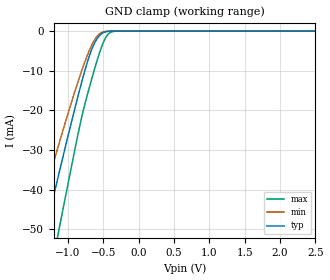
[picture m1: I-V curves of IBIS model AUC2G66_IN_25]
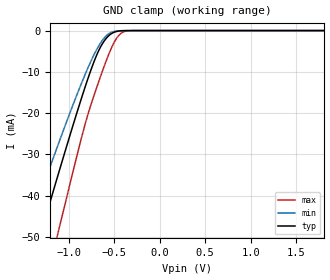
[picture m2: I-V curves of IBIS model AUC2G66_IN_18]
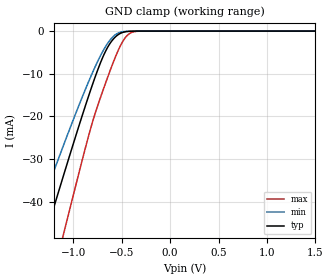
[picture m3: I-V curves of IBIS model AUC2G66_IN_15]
| TEXAS INSTRUMENTS INCORPORATED
| Standard Linear and Logic Group
| IBIS Model of SN74AUC2G66
| DUAL BILATERAL ANALOG SWITCH
| This file contains package information for the following:
|  SOT 8-pin (DCT) package as [Component] AUC2G66_DCT
|  TSSOP 8-pin (DCU) package as [Component] AUC2G66_DCU
|  NanoStar WCSP 8-pin (YEP) package as [Component] AUC2G66_YEP
|  NanoFree WCSP 8-pin (YZP) package as [Component] AUC2G66_YZP
| This device can be powered at the following Vccs:
|  2.5 volt Vcc
|  1.8 volt Vcc
|  1.5 volt Vcc
|  1.2 volt Vcc
| This file provides unique models under the [Model Selector] for each Vcc.
| For operation at a specific Vcc, select the appropriate model after each
| [Model Selector] keyword.
[IBIS Ver]   3.2
[Comment char]  |_char
[File Name]   sn74auc2g66.ibs
[File Rev]   1.3 | x_die
[Date]   May 25, 2004
[Source]   Data created from TI-SPICE simulations at TI-SLL.
[Notes]   The following is an IBIS list for the AUC2G66.
   Please contact sllibis@ti.com with questions and
   comments concerning SLL IBIS models.
   - FILE REV HISTORY
   - 1.3 YEP and YZP packages added on 05/25/04
   - Non-monotonic data due to FET characteristics.
   - The series-switch models may generate errors
   "Series_MOSFET has Decreasing Current" if checked with
   IBISCHK version 3.2.8 or older. These errors are due to
   a bug in the older versions of IBISCHK parsers.
[Disclaimer] Property of Texas Instruments Incorporated. Unauthorized
   reproduction and/or distribution is strictly prohibited.
   This product is protected under copyright law.
   Created 2003,(C) Copyright 2003, Texas Instruments
   Incorporated, All Rights Reserved
   UNLESS THERE IS A SIGNED, WRITTEN AGREEMENT TO THE
   CONTRARY, TEXAS INSTRUMENTS (TI) IS PROVIDING THE IBIS
   MODELS AND WITHOUT ANY WARRANTY, EXPRESSED OR
   IMPLIED. TI assumes no liability for:
   1) the accuracy of the IBIS models provided to your
   company;
   2) the proper functioning of these IBIS Models in your
   design or for any resulting applications; or
   3) infringement of patents, copyrights or intellectual
   property rights resulting from your use of these IBIS
   models.
   TI provides IBIS Models as a service to our customers.
   You and your company shall not distribute, sell or give
   these models to anyone else without prior written
   permission from TI.
   TI reserves the right to make changes to our products or
   to discontinue any semiconductor product or service
   without notice, and advises our customers to obtain the
   latest version of relevant information to verify, before
   placing orders, that the information being relied on is
   current.
   Please be aware that your receipt and use of the IBIS
   information provided shall serve as acceptance of these
   terms and conditions. If you do not accept these terms,
   you should return or destroy the IBIS models and any
   other accompanying information immediately.
| Component AUC2G66_DCT 8-pin SOT
[Component]   AUC2G66_DCT
[Manufacturer]   Texas Instruments, Inc.
[Package]
|   typ   min   max
R_pkg   2.900e-02   2.800e-02   3.100e-02
L_pkg   1.796e-09   1.666e-09   1.924e-09
C_pkg   2.310e-13   2.210e-13   2.420e-13
[Pin]   signal_name   model_name   R_pin   L_pin   C_pin
1   1A   AUC2G66_IO   3.100e-02   1.894e-09   2.230e-13
2   1B   AUC2G66_IO   2.800e-02   1.697e-09   2.370e-13
3   2C   AUC2G66_IN   3.000e-02   1.722e-09   2.390e-13
4   GND   GND   3.000e-02   1.861e-09   2.210e-13
5   2A   AUC2G66_IO   2.800e-02   1.924e-09   2.280e-13
6   2B   AUC2G66_IO   2.900e-02   1.736e-09   2.420e-13
7   1C   AUC2G66_IN   2.800e-02   1.666e-09   2.360e-13
8   VCC   POWER   3.000e-02   1.871e-09   2.220e-13
| Component AUC2G66_DCU 8-pin TSSOP
[Component]   AUC2G66_DCU
[Manufacturer]   Texas Instruments, Inc.
[Package]
|   typ   min   max
R_pkg   1.400e-02   1.300e-02   1.500e-02
L_pkg   1.289e-09   1.025e-09   2.014e-09
C_pkg   1.360e-13   6.600e-14   2.940e-13
[Pin]   signal_name   model_name   R_pin   L_pin   C_pin
1   1A   AUC2G66_IO   1.400e-02   1.387e-09   1.760e-13
2   1B   AUC2G66_IO   1.300e-02   1.026e-09   6.600e-14
3   2C   AUC2G66_IN   1.300e-02   1.032e-09   6.700e-14
4   GND   GND   1.500e-02   2.014e-09   2.940e-13
5   2A   AUC2G66_IO   1.400e-02   1.412e-09   1.780e-13
6   2B   AUC2G66_IO   1.300e-02   1.030e-09   6.600e-14
7   1C   AUC2G66_IN   1.300e-02   1.025e-09   6.600e-14
8   VCC   POWER   1.400e-02   1.386e-09   1.760e-13
| Component AUC2G66_YEP 8-pin NanoStar WCSP
[Component]   AUC2G66_YEP
[Manufacturer]   Texas Instruments, Inc.
[Package]
|   typ   min   max
R_pkg   0.001   0.001   0.001
L_pkg   0.021nH   0.021nH   0.021nH
C_pkg   0.043pF   0.042pF   0.044pF
[Pin]   signal_name   model_name   R_pin   L_pin   C_pin
1   1A   AUC2G66_IO   0.046   2.861nH   0.321pF
2   1B   AUC2G66_IO   0.037   2.437nH   0.286pF
3   2C   AUC2G66_IN   0.034   2.419nH   0.286pF
4   GND   GND   0.043   2.784nH   0.321pF
5   2A   AUC2G66_IO   0.043   2.784nH   0.321pF
6   2B   AUC2G66_IO   0.035   2.420nH   0.286pF
7   1C   AUC2G66_IN   0.037   2.437nH   0.286pF
8   VCC   POWER   0.046   2.860nH   0.321pF
| Component AUC2G66_YZP 8-pin NanoFree WCSP
[Component]   AUC2G66_YZP
[Manufacturer]   Texas Instruments, Inc.
[Package]
|   typ   min   max
R_pkg   0.001   0.001   0.001
L_pkg   0.021nH   0.021nH   0.021nH
C_pkg   0.043pF   0.042pF   0.044pF
[Pin]   signal_name   model_name   R_pin   L_pin   C_pin
1   1A   AUC2G66_IO   0.046   2.861nH   0.321pF
2   1B   AUC2G66_IO   0.037   2.437nH   0.286pF
3   2C   AUC2G66_IN   0.034   2.419nH   0.286pF
4   GND   GND   0.043   2.784nH   0.321pF
5   2A   AUC2G66_IO   0.043   2.784nH   0.321pF
6   2B   AUC2G66_IO   0.035   2.420nH   0.286pF
7   1C   AUC2G66_IN   0.037   2.437nH   0.286pF
8   VCC   POWER   0.046   2.860nH   0.321pF
[Series Switch Groups]
| Function Group States
On  1 /   | 1A<->1B(1C=HIGH)
On  2 /   | 2A<->2B(2C=HIGH)
On  1 2 /   | Both ON(1C=HIGH,2C=HIGH)
[Series Pin Mapping]   pin_2   model_name   function_table_group
1   2   AUC2G66_IO_25_S   1
| 1   2   AUC2G66_IO_18_S   1
| 1   2   AUC2G66_IO_15_S   1
| 1   2   AUC2G66_IO_12_S   1
5   6   AUC2G66_IO_25_S   2
| 5   6   AUC2G66_IO_18_S   2
| 5   6   AUC2G66_IO_15_S   2
| 5   6   AUC2G66_IO_12_S   2
| Model AUC2G66_IN
[Model Selector]   AUC2G66_IN
AUC2G66_IN_25   2.5 volt Vcc
AUC2G66_IN_18   1.8 volt Vcc
AUC2G66_IN_15   1.5 volt Vcc
AUC2G66_IN_12   1.2 volt Vcc
| Model AUC2G66_IO
[Model Selector]   AUC2G66_IO
AUC2G66_IO_25   2.5 volt Vcc
AUC2G66_IO_18   1.8 volt Vcc
AUC2G66_IO_15   1.5 volt Vcc
AUC2G66_IO_12   1.2 volt Vcc
| Model AUC2G66_IO_S
[Model Selector]   AUC2G66_IO_S
AUC2G66_IO_25_S   2.5 volt Vcc_S
AUC2G66_IO_18_S   1.8 volt Vcc_S
AUC2G66_IO_15_S   1.5 volt Vcc_S
AUC2G66_IO_12_S   1.2 volt Vcc_S
[Model]   AUC2G66_IO_25_S
Model_type  Series_switch
| variable   typ   min   max
C_comp   0   0   0
[Temperature Range]   40   100   -40
| Ambient temperature   25   85   -40
[Voltage range]   2.5   2.3   2.7
[On]
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[Off]
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[Model]   AUC2G66_IO_18_S
Model_type  Series_switch
| variable   typ   min   max
C_comp   0   0   0
[Temperature Range]   40   100   -40
| Ambient temperature   25   85   -40
[Voltage range]   1.8   1.65   1.95
[On]
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[Off]
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[Model]   AUC2G66_IO_15_S
Model_type  Series_switch
| variable   typ   min   max
C_comp   0   0   0
[Temperature Range]   40   100   -40
| Ambient temperature   25   85   -40
[Voltage range]   1.5   1.4   1.6
[On]
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[Off]
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[Model]   AUC2G66_IO_12_S
Model_type  Series_switch
| variable   typ   min   max
C_comp   0   0   0
[Temperature Range]   40   100   -40
| Ambient temperature   25   85   -40
[Voltage range]   1.2   1.1   1.3
[On]
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[Off]
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| Models and submodels in the file (12): AUC2G66_IN_25 (Input), AUC2G66_IN_18 (Input), AUC2G66_IN_15 (Input), AUC2G66_IN_12 (Input), AUC2G66_IO_25_S (Series_switch), AUC2G66_IO_25 (Terminator), AUC2G66_IO_18_S (Series_switch), AUC2G66_IO_18 (Terminator), AUC2G66_IO_15_S (Series_switch), AUC2G66_IO_15 (Terminator), AUC2G66_IO_12_S (Series_switch), AUC2G66_IO_12 (Terminator)
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[Model]   AUC2G66_IN_25
Model_type  Input
Vinl=0.7
Vinh=1.7
| variable   typ   min   max
C_comp   1.89pF   1.48pF   2.30pF
[Temperature Range]   40   100   -40
| Ambient temperature   25   85   -40
[Voltage range]   2.5   2.3   2.7
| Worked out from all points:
|   GND clamp passes 1 mA (typ) near -0.55 V on its own axis
[GND Clamp]
| AUC2G66_IN_25
|   Voltage   I(typ)   I(min)   I(max)
-2.7V     -157mA     -130.3mA   -191.7mA
-1.47V    -61.86mA   -49.74mA   -81.22mA
-1.32V    -50.42mA   -40.3mA    -67.62mA
-1.15V    -37.6mA    -29.81mA   -52.18mA
-1.11V    -34.62mA   -27.39mA   -48.55mA
-855mV    -16.2mA    -12.62mA   -25.76mA
-740mV    -8.694mA   -6.762mA   -17.01mA
-635mV    -3.435mA   -2.557mA   -10.25mA
-530mV    -751.7uA   -416uA     -4.264mA
-440mV    -95.44uA   -46.04uA   -977.4uA
-335mV    -4.571uA   -2.694uA   -44.25uA
2.5V      313.9pA    402pA      470.4pA
[Model]   AUC2G66_IN_18
Model_type  Input
Vinl=0.5775
Vinh=1.2675
| variable   typ   min   max
C_comp   1.97pF   1.57pF   2.31pF
[Temperature Range]   40   100   -40
| Ambient temperature   25   85   -40
[Voltage range]   1.8   1.65   1.95
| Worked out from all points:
|   GND clamp passes 1 mA (typ) near -0.55 V on its own axis
[GND Clamp]
| AUC2G66_IN_18
|   Voltage   I(typ)   I(min)   I(max)
-2.7V     -157mA     -130.3mA   -191.7mA
-1.485V   -63.01mA   -50.7mA    -82.58mA
-1.435V   -59.19mA   -47.53mA   -78.05mA
-1.295V   -48.52mA   -38.74mA   -65.35mA
-1.13V    -36.11mA   -28.6mA    -50.37mA
-1.09V    -33.13mA   -26.19mA   -46.74mA
-735mV    -8.396mA   -6.53mA    -16.67mA
-640mV    -3.626mA   -2.718mA   -10.56mA
-540mV    -904.5uA   -517.4uA   -4.766mA
-445mV    -108.7uA   -52.4uA    -1.09mA
-345mV    -6.234uA   -3.562uA   -63.03uA
1.8V      203.2pA    298.4pA    235.5pA
[Model]   AUC2G66_IN_15
Model_type  Input
Vinl=0.49
Vinh=1.04
| variable   typ   min   max
C_comp   2.01pF   1.62pF   2.32pF
[Temperature Range]   40   100   -40
| Ambient temperature   25   85   -40
[Voltage range]   1.5   1.4   1.6
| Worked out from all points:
|   GND clamp passes 1 mA (typ) near -0.55 V on its own axis
[GND Clamp]
| AUC2G66_IN_15
|   Voltage   I(typ)   I(min)   I(max)
-2.7V     -157mA     -130.3mA   -191.7mA
-1.45V    -60.33mA   -48.48mA   -79.41mA
-1.405V   -56.89mA   -45.63mA   -75.33mA
-1.27V    -46.63mA   -37.19mA   -63.08mA
-1.11V    -34.62mA   -27.39mA   -48.55mA
-1.075V   -32.02mA   -25.29mA   -45.38mA
-740mV    -8.694mA   -6.762mA   -17.01mA
-640mV    -3.626mA   -2.718mA   -10.56mA
-540mV    -904.5uA   -517.4uA   -4.766mA
-445mV    -108.7uA   -52.4uA    -1.09mA
-340mV    -5.34uA    -3.098uA   -52.88uA
1.5V      165.9pA    259.7pA    172.1pA
